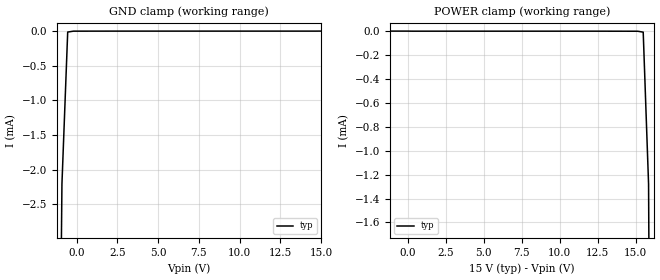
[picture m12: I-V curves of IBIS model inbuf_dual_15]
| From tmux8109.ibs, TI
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| inbuf_dual_15
[Model]   inbuf_dual_15
Model_type   Input
Vinl = 1.3
Vinh = 0.8
|   typ   min   max
C_comp   4.014581e-13   NA   NA
[Voltage Range]   15   NA   NA
[Temperature Range]   27   NA   NA
[Power Clamp Reference]   15   NA   NA
[GND Clamp Reference]   0   NA   NA
[GND Clamp]
|   Voltage   I(typ)   I(min)   I(max)
-20V      -547.9mA   NA         NA
-1.263V   -10.94mA   NA         NA
-909.1mV  -2.21mA    NA         NA
-555.6mV  -13.03uA   NA         NA
-202mV    -42.85nA   NA         NA
15V       1.003uA    NA         NA
[POWER Clamp]
|   Voltage   I(typ)   I(min)   I(max)
-5V       1.33uA     NA         NA
15.15V    -31.49nA   NA         NA
15.51V    -7.666uA   NA         NA
15.86V    -1.279mA   NA         NA
16.21V    -9.608mA   NA         NA
30V       -403.9mA   NA         NA
